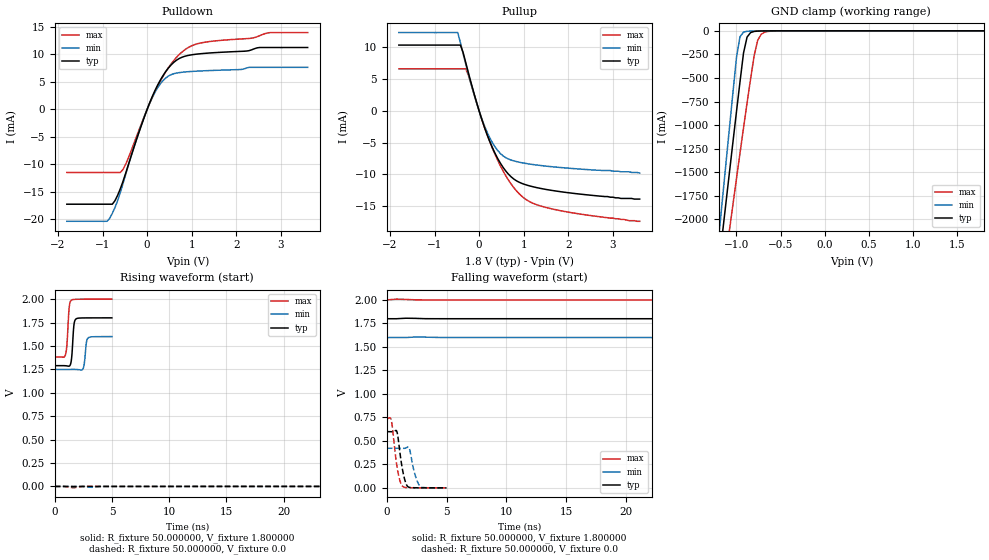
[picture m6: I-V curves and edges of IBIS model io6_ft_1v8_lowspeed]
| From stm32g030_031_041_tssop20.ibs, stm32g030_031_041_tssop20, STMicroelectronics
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|   Model io6_ft_1v8_lowspeed
[Model]  io6_ft_1v8_lowspeed
Model_type I/O
Polarity   Non-Inverting
Enable   Active-Low
Vinl =   0.540000V
Vinh =   1.260000V
Vmeas =  0.900000V
Cref =   30.000000pF
Rref =   100.000000M
Vref =   0.0V
C_comp   1.277600pF   1.236700pF   1.315100pF
[Temperature Range]   25.000000   -40.000000   0.125000k
[Pullup Reference]   1.800000V   1.600000V   2.000000V
[Pulldown Reference]   0.0V   0.0V   0.0V
[POWER Clamp Reference]   1.800000V   1.600000V   2.000000V
[GND Clamp Reference]   0.0V   0.0V   0.0V
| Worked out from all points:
|   slope of the pulldown table from 0 to 0.27 V, typ, clamps not added: 54.7 ohm
|   slope of the pullup table from 0 to 0.27 V, typ, clamps not added: 50.6 ohm
|   GND clamp passes 1 mA (typ) near -0.66 V on its own axis
|   rising waveform, R_fixture 50.000000, V_fixture 1.800000: 20-80 % time 165ps typ, 169ps min, 180ps max; typ from 1.29 V to 1.8 V
|   rising waveform, R_fixture 50.000000, V_fixture 0.0: 20-80 % time 98.3ns typ, 95.5ns min, 113ns max; typ from 0 V to 0.598 V
|   falling waveform, R_fixture 50.000000, V_fixture 1.800000: 20-80 % time 97.2ns typ, 101ns min, 95.8ns max; typ from 1.8 V to 1.29 V
|   falling waveform, R_fixture 50.000000, V_fixture 0.0: 20-80 % time 437ps typ, 477ps min, 447ps max; typ from 0.598 V to 0 V
[Pulldown]
|Voltage   I(typ)   I(min)   I(max)
-1.8V     -17.22mA   -20.33mA   -11.45mA
-900mV    -17.22mA   -20.33mA   -11.45mA
-720mV    -16.58mA   -17.82mA   -11.45mA
-600mV    -14.41mA   -15.08mA   -11.45mA
-480mV    -11.58mA   -11.79mA   -9.954mA
0V        10fA       11fA       0A
240mV     4.49mA     3.999mA    4.291mA
480mV     7.563mA    6.085mA    7.612mA
780mV     9.487mA    6.76mA     10.43mA
1.14V     10.08mA    6.976mA    11.96mA
2.76V     11.26mA    7.652mA    13.98mA
3.6V      11.26mA    7.652mA    13.98mA
[Pullup]
|Voltage   I(typ)   I(min)   I(max)
-1.8V     10.37mA    12.35mA    6.631mA
-480mV    10.37mA    12.35mA    6.631mA
-420mV    10.37mA    10.77mA    6.631mA
-300mV    7.616mA    7.38mA     6.631mA
-240mV    5.996mA    5.774mA    5.613mA
-60mV     1.422mA    1.342mA    1.368mA
120mV     -2.605mA   -2.366mA   -2.563mA
360mV     -6.731mA   -5.708mA   -6.907mA
600mV     -9.499mA   -7.385mA   -10.25mA
960mV     -11.43mA   -8.172mA   -13.47mA
1.32V     -12.13mA   -8.557mA   -14.86mA
3.6V      -13.9mA    -9.8mA     -17.4mA
[GND_clamp]
|Voltage   I(typ)   I(min)   I(max)
-1.8V     -7.471A    -7.973A    -7.298A
-1.2V     -2.489A    -2.18A     -2.954A
-1.16V    -2.16A     -1.797A    -2.674A
-1.08V    -1.505A    -1.034A    -2.118A
-1V       -857.9mA   -283.1mA   -1.568A
-960mV    -540.4mA   -62.14mA   -1.296A
-920mV    -234.4mA   -13.75mA   -1.028A
-880mV    -66.29mA   -4.855mA   -765.3mA
-800mV    -6.505mA   -2.056mA   -266mA
-760mV    -3.074mA   -1.45mA    -100.4mA
-680mV    -1.215mA   -557.1uA   -14.19mA
1.8V      0A         0A         0A
[POWER_clamp]
|Voltage   I(typ)   I(min)   I(max)
-1.8V     0A         0A         0A
0V        0A         0A         0A
[Ramp]
| variable   typ   min   max
dV/dt_r  0.35701/98.22318n   0.25147/95.47453n   0.43805/0.11268u
dV/dt_f  0.30018/97.04176n   0.211/0.10048u   0.36564/95.79000n
R_load = 50.000000
[Rising Waveform]
R_fixture= 50.000000
V_fixture= 1.800000
V_fixture_min= 1.600000
V_fixture_max= 2.000000
|time   V(typ)   V(min)   V(max)
0s        1.29V      1.249V     1.383V
940.9ps   1.289V     1.249V     1.409V
1.061ns   1.287V     1.249V     1.515V
1.261ns   1.285V     1.249V     1.913V
1.421ns   1.329V     1.249V     1.985V
1.672ns   1.722V     1.249V     1.997V
1.852ns   1.788V     1.249V     1.998V
2.482ns   1.799V     1.26V      2V
2.893ns   1.8V       1.583V     2V
4.985ns   1.8V       1.6V       2V
[Rising Waveform]
R_fixture= 50.000000
V_fixture= 0.0
V_fixture_min= 0.0
V_fixture_max= 0.0
|time   V(typ)   V(min)   V(max)
0s        -200.9nV   1.601uV    485nV
1.602ns   -1.318mV   -4.562uV   -15.15mV
36.84ns   156.4uV    -27.8uV    8.957mV
63.26ns   28.2mV     72.48uV    79.22mV
92.09ns   136mV      25.52mV    210.1mV
144.1ns   360.3mV    187.2mV    448.3mV
171.4ns   443.2mV    264.4mV    538mV
204.2ns   509.5mV    330.6mV    614.7mV
274.7ns   574.3mV    397.8mV    698.8mV
398.8ns   597.9mV    421.2mV    736.3mV
[Falling Waveform]
R_fixture= 50.000000
V_fixture= 1.800000
V_fixture_min= 1.600000
V_fixture_max= 2.000000
|time   V(typ)   V(min)   V(max)
0s        1.8V       1.6V       2V
52.05ns   1.8V       1.6V       1.983V
68.07ns   1.798V     1.6V       1.943V
92.09ns   1.774V     1.6V       1.851V
118.5ns   1.707V     1.599V     1.73V
147.3ns   1.602V     1.587V     1.605V
194.6ns   1.441V     1.511V     1.484V
233ns     1.37V      1.418V     1.438V
288.3ns   1.322V     1.317V     1.406V
398.8ns   1.29V      1.249V     1.383V
[Falling Waveform]
R_fixture= 50.000000
V_fixture= 0.0
V_fixture_min= 0.0
V_fixture_max= 0.0
|time   V(typ)   V(min)   V(max)
0s        597.9mV    421.2mV    736.3mV
390.4ps   597.4mV    421.3mV    710.6mV
830.8ps   603.2mV    421.5mV    247.8mV
1.081ns   394.7mV    421.5mV    84.11mV
1.321ns   190.5mV    420.9mV    17.3mV
1.572ns   58.37mV    422.8mV    3.714mV
1.862ns   6.504mV    427.8mV    1.544mV
2.362ns   1.256mV    141mV      603.4uV
2.823ns   477.3uV    11.23mV    326.6uV
4.985ns   -200.9nV   1.601uV    485nV
